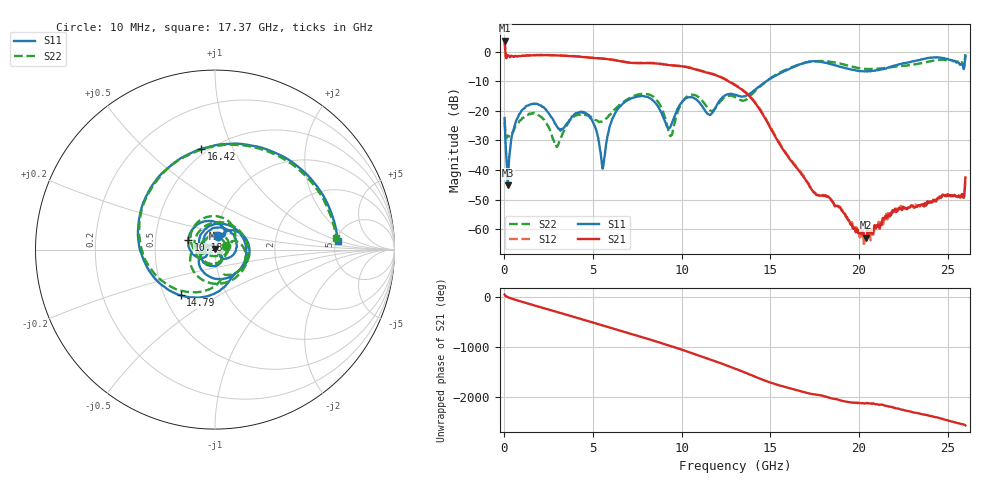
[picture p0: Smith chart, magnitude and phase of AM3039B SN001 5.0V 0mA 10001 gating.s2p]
!Agilent Technologies,E8364B,MY43040894,A.07.50.67
!Agilent E8364B: A.07.50.67
!Date: Tuesday, June 28, 2016 08:07:27
!Correction: S11(Full 2 Port(1,2))
!S21(Full 2 Port(1,2))
!S12(Full 2 Port(1,2))
!S22(Full 2 Port(1,2))
!S2P File: Measurements: S11, S21, S12, S22:
# Hz S  dB  R 50
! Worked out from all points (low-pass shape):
!   1601 points, 10 MHz to 26 GHz, reference 50 ohm
!   highest |S21| = 3.68 dB at 10 MHz (marker M1); lowest = -62.8 dB at 20.41 GHz (marker M2)
!   |S21| within 3 dB of the highest: start of sweep to 44.2 MHz
!   lowest |S11| = -45.2 dB at 188.7 MHz (marker M3), VSWR 1.01, Z = 49.7 + j0.482 ohm
!   |S11| at or under -10 dB: start of sweep to 14.78 GHz
!   |S22| runs from -32.2 to -0.9 dB; largest |S21 - S12| = 0.025
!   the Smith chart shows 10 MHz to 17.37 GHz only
!   S11 on the Smith chart (normalised r, x): 10 MHz: 1.03, +0.15; 10.18 GHz: 0.74, +0.08; 14.79 GHz: 0.61, -0.34; 16.42 GHz: 0.46, +0.76; 17.37 GHz: 5.16, +0.97
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1e7  -22.45 75.7  3.68 40.8  3.74 41.6  -23.81 16.7
1.886812e8  -45.16 118.7  -1.24 -10.6  -1.19 -10.5  -28.34 -60.1
1.634375e9  -17.54 53.5  -1.25 -169.9  -1.21 -169.7  -20.70 56.3
2.673975e9  -22.30 -41.0  -1.26 83.7  -1.18 83.9  -28.26 -49.8
3.502406e9  -24.40 -49.3  -1.45 -1.2  -1.40 -1.1  -25.11 -45.1
4.347081e9  -20.45 -122.8  -1.79 -88.8  -1.76 -88.7  -21.15 -148.9
5.971456e9  -24.67 -165.3  -2.69 100.9  -2.61 101.2  -21.29 -115.2
6.994812e9  -16.32 66.7  -3.73 -5.7  -3.66 -5.3  -15.92 69.7
8.684162e9  -18.76 -141.3  -4.10 173.8  -4.02 174.4  -17.09 -166.6
1.017859e10  -15.99 160.5  -5.14 3.9  -5.05 4.4  -15.81 145.3
1.160804e10  -21.37 59.9  -7.39 -168.6  -7.28 -167.9  -19.91 24.4
1.3005e10  -14.55 -27.4  -11.34 8.4  -11.18 9.4  -15.35 -52.5
1.479181e10  -9.93 -126.8  -23.46 116.9  -23.15 117.5  -9.96 -138.4
1.641619e10  -4.94 98.0  -38.77 -53.2  -38.48 -52.9  -4.80 90.6
1.734208e10  -3.30 7.5  -46.64 -135.8  -46.52 -136.2  -3.38 8.5
1.737457e10  -3.29 4.2  -46.95 -137.6  -46.79 -137.4  -3.35 5.6
1.847914e10  -4.37 -103.0  -50.44 134.5  -50.42 135.5  -3.51 -93.3
2.041215e10  -6.70 106.5  -62.84 42.6  -60.88 44.5  -5.91 116.7
2.167916e10  -5.34 20.4  -55.65 -24.1  -54.30 -26.6  -5.39 27.0
2.317359e10  -3.09 -92.0  -52.38 -147.5  -51.76 -147.6  -4.29 -81.6
2.427816e10  -1.98 178.4  -49.94 125.5  -50.03 128.8  -3.01 -165.5
2.6e10  -1.67 -17.0  -42.48 -41.7  -42.32 -38.5  -0.89 14.6
